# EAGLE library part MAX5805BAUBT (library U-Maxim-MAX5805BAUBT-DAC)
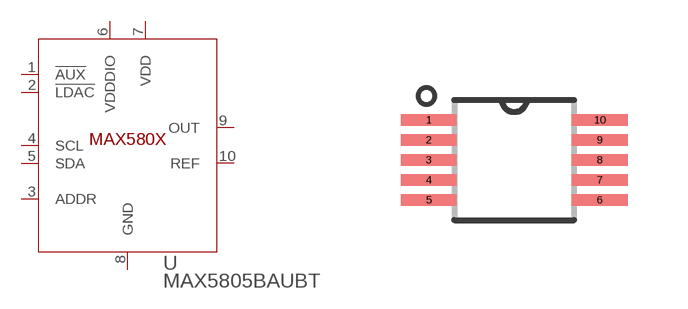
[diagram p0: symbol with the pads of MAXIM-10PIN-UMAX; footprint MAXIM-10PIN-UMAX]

Designator prefix U

## MAX5805BAUBT (DESCRIPTION: Data acquisition IC - DA converter _DAC_ Maxim Integrated MAX5805BAUB+ uMAX 10; DIGI-KEY_PART_NUMBER: MAX5805BAUB+-ND; DIGI-KEY_PURCHASE_URL: https://www.digikey.com/product-detail/en/maxim-integrated/MAX5805BAUB-/MAX5805BAUB--ND/4271373?utm_source=snapeda&utm_medium=aggregator&utm_campaign=symbol; MF: Maxim Integrated; MP: MAX5805BAUB+; PACKAGE: uMAX-10 Maxim)  [MAXIM-10PIN-UMAX]
1  !AUX  in
2  !LDAC  in
3  ADDR  in
4  SCL  in
5  SDA
6  VDDDIO  pwr
7  VDD  pwr
8  GND  pwr
9  OUT  out
10  REF

## Footprint MAXIM-10PIN-UMAX (pad centres in mm)
smd 1.4 x 0.28: 1 -2.14,1; 2 -2.14,0.5; 3 -2.14,0; 4 -2.14,-0.5; 5 -2.14,-1; 6 2.14,-1; 7 2.14,-0.5; 8 2.14,0; 9 2.14,0.5; 10 2.14,1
